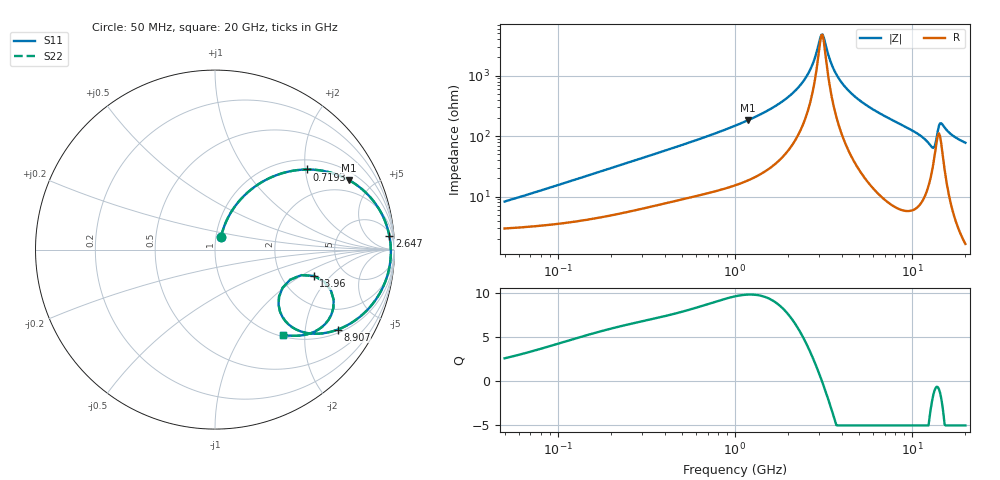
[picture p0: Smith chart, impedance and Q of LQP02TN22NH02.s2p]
!Murata Part Number: LQP02TN22NH02
!These Parameters are Measured in Series Mode Connection
!  o--[Z]--o
!Port1  Port2
!  o-------o
!Freq. Start=50[MHz] Stop=20[GHz], 401[Steps]
# Hz S RI R 50
!Freq.(Hz) S11(Real) S11(Imag) S21(Real) S21(Imag) S12(Real) S12(Imag) S22(Real) S22(Imag)
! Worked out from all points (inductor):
!   401 points, 50 MHz to 20 GHz, reference 50 ohm
!   read as one part in series: L = 24.3 nH near 60.75 MHz
!   highest Q = 9.82 at 1.179 GHz (marker M1), where L = 24.5 nH
!   self-resonance near 3.075 GHz
!   S11 on the Smith chart (normalised r, x): 50 MHz: 1.06, +0.16; 719.3 MHz: 1.23, +2.04; 2.647 GHz: 8, +23; 8.907 GHz: 1.12, -2.98; 13.96 GHz: 3.02, -1.31; 20 GHz: 1.03, -1.55
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5e7  0.0344 0.0727  0.9656 -0.0727  0.9656 -0.0727  0.0344 0.0727
1.364002e8  0.074 0.1811  0.926 -0.1811  0.926 -0.1811  0.074 0.1811
3.721004e8  0.2505 0.3697  0.7495 -0.3697  0.7495 -0.3697  0.2505 0.3697
7.192613e8  0.5123 0.4463  0.4877 -0.4463  0.4877 -0.4463  0.5123 0.4463
1e9  0.6713 0.4207  0.3287 -0.4207  0.3287 -0.4207  0.6713 0.4207
1.179116e9  0.7472 0.3867  0.2528 -0.3867  0.2528 -0.3867  0.7472 0.3867
1.962148e9  0.9235 0.2091  0.0765 -0.2091  0.0765 -0.2091  0.9235 0.2091
2.647493e9  0.9718 0.0745  0.0282 -0.0745  0.0282 -0.0745  0.9718 0.0745
2.728004e9  0.9743 0.0605  0.0257 -0.0605  0.0257 -0.0605  0.9743 0.0605
3.029571e9  0.9794 0.0109  0.0206 -0.0109  0.0206 -0.0109  0.9794 0.0109
3.121702e9  0.9798 -0.00336  0.0202 0.00336  0.0202 0.00336  0.9798 -0.00336
3.572216e9  0.9764 -0.0679  0.0236 0.0679  0.0236 0.0679  0.9764 -0.0679
4.149438e9  0.9618 -0.1396  0.0382 0.1396  0.0382 0.1396  0.9618 -0.1396
5.273168e9  0.9134 -0.2516  0.0866 0.2516  0.0866 0.2516  0.9134 -0.2516
7.442007e9  0.7831 -0.3928  0.2169 0.3928  0.2169 0.3928  0.7831 -0.3928
8.907419e9  0.6826 -0.4461  0.3174 0.4461  0.3174 0.4461  0.6826 -0.4461
1.131968e10  0.4937 -0.4606  0.5063 0.4606  0.5063 0.4606  0.4937 -0.4606
1.276073e10  0.3619 -0.3446  0.6381 0.3446  0.6381 0.3446  0.3619 -0.3446
1.396067e10  0.5503 -0.1463  0.4497 0.1463  0.4497 0.1463  0.5503 -0.1463
1.482269e10  0.6595 -0.3245  0.3405 0.3245  0.3405 0.3245  0.6595 -0.3245
1.597544e10  0.5774 -0.4445  0.4226 0.4445  0.4226 0.4445  0.5774 -0.4445
2e10  0.379 -0.4746  0.621 0.4746  0.621 0.4746  0.379 -0.4746
